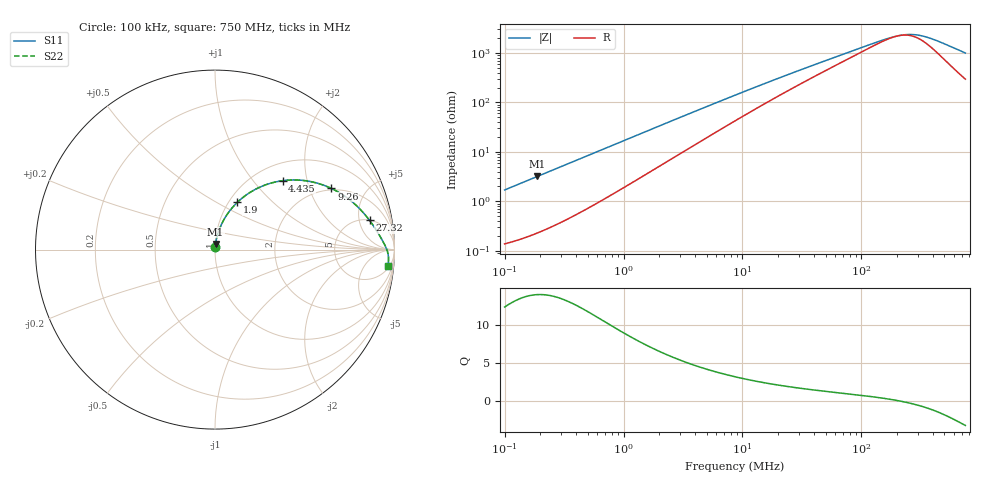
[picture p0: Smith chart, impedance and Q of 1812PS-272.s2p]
# MHz S MA R 50
!Freq  MagS11  AngS11  MagS21  AngS21  MagS12  AngS12  MagS22  AngS22
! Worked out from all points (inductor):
!   801 points, 100 kHz to 750 MHz, reference 50 ohm
!   read as one part in series: L = 2.7 uH near 104.6 kHz
!   highest Q = 13.9 at 188.8 kHz (marker M1), where L = 2.69 uH
!   self-resonance near 206.5 MHz
!   S11 on the Smith chart (normalised r, x): 100 kHz: 1.00, +0.03; 1.9 MHz: 1.10, +0.63; 4.435 MHz: 1.33, +1.43; 9.26 MHz: 1.93, +2.84; 27.32 MHz: 5.06, +7.11; 750 MHz: 7, -19
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0.1  0.01697 84.4  0.9985 -1.0  0.9985 -1.0  0.01697 84.4
0.1888418  0.03196 84.1  0.9972 -1.8  0.9972 -1.8  0.03196 84.1
0.4457309  0.07481 81.0  0.9911 -4.3  0.9911 -4.3  0.07481 81.0
1.040408  0.1697 73.8  0.9664 -9.7  0.9664 -9.7  0.1697 73.8
1.900073  0.2916 64.7  0.9141 -16.8  0.9141 -16.8  0.2916 64.7
1.964725  0.3 64.1  0.9097 -17.2  0.9097 -17.2  0.3 64.1
2.902924  0.408 55.9  0.8419 -23.7  0.8419 -23.7  0.408 55.9
4.435076  0.5377 45.6  0.7323 -31.6  0.7323 -31.6  0.5377 45.6
6.128751  0.6323 37.4  0.6286 -37.7  0.6286 -37.7  0.6323 37.4
8.660254  0.7182 29.2  0.5118 -43.2  0.5118 -43.2  0.7182 29.2
9.259629  0.7326 27.7  0.4896 -44.1  0.4896 -44.1  0.7326 27.7
15.29557  0.8173 18.3  0.34 -48.8  0.34 -48.8  0.8173 18.3
27.31774  0.8764 10.7  0.214 -49.5  0.214 -49.5  0.8764 10.7
38.60143  0.8995 7.6  0.1611 -47.7  0.1611 -47.7  0.8995 7.6
72.89563  0.9289 3.8  0.09525 -39.9  0.09525 -39.9  0.9289 3.8
170.1501  0.9534 0.6  0.04777 -12.2  0.04777 -12.2  0.9534 0.6
203.3919  0.9571 0.0  0.04293 -1.1  0.04293 -1.1  0.9571 0.0
235.1274  0.9598 -0.4  0.04085 9.6  0.04085 9.6  0.9598 -0.4
268.8  0.962 -0.8  0.04065 20.3  0.04065 20.3  0.962 -0.8
310.7413  0.9641 -1.3  0.0425 31.6  0.0425 31.6  0.9641 -1.3
415.2776  0.9672 -2.4  0.05255 50.2  0.05255 50.2  0.9672 -2.4
750  0.9672 -5.3  0.0966 67.5  0.0966 67.5  0.9672 -5.3
